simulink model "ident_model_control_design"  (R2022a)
settings: Solver=VariableStepAuto  StartTime=0.0  StopTime=tfin  RelTol=1e-3
undefined symbols (not defined in the file or in its folder): magnitude
libraries: cstblocks x5, mpclib x2, slpidlib x1, ctrlSharedLib x1

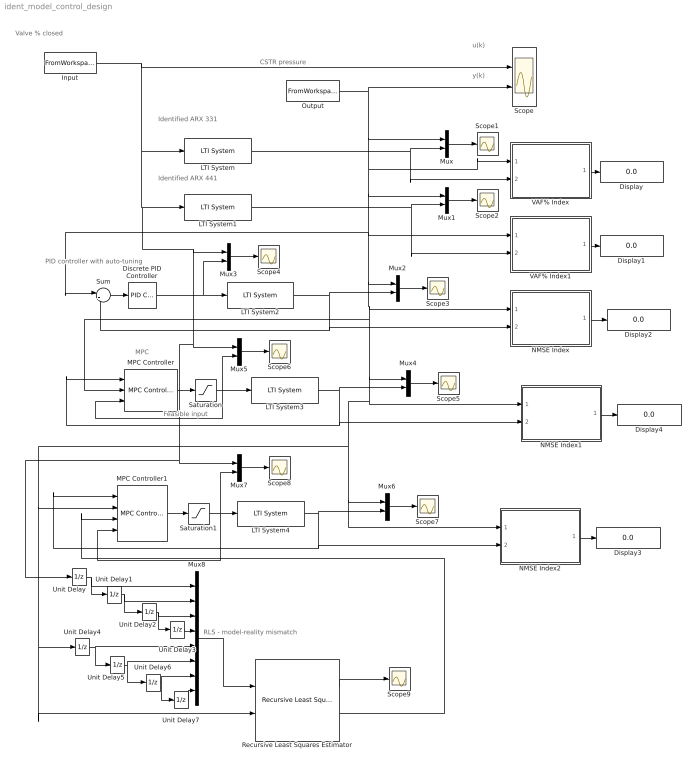
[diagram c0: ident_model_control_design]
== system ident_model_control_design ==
  note: RLS - model-reality mismatch
  note: Feasible input
  note: PID controller with auto-tuning
  note: Identified ARX 441
  note: Identified ARX 331
  note: y(k)
  note: u(k)
  note: CSTR pressure
  note: Valve % closed
  note: MPC
  Discrete PID Controller : slpidlib/PID Controller  Controller=PID  Form=Parallel  TimeDomain=Discrete-time  UseExternalTs=off  SampleTime=5  IntegratorMethod=Forward Euler  FilterMethod=Backward Euler  ControllerParametersSource=internal  P=34.9781098991711  I=1.59717324757153  UseKiTs=off  D=0  N=100  UseFilter=on  TunerSelectOption=Transfer Function Based (PID Tuner App)  InitialConditionSource=internal  InitialConditionForIntegrator=0  InitialConditionForFilter=0  DifferentiatorICPrevScaledInput=0  ExternalReset=none  TrackingMode=off  Kt=1  LimitOutput=off  SatLimitsSource=internal  UpperSaturationLimit=inf  LowerSaturationLimit=-inf  LinearizeAsGain=off  AntiWindupMode=none  Kb=1  POutMin=[]  POutMax=[]  IOutMin=[]  IOutMax=[]  DOutMin=[]  DOutMax=[]  NOutMin=[]  NOutMax=[]  SumOutMin=[]  SumOutMax=[]  SaturationOutMin=[]  SaturationOutMax=[]  PParamMin=[]  PParamMax=[]  IParamMin=[]  IParamMax=[]  DParamMin=[]  DParamMax=[]  NParamMin=[]  NParamMax=[]  KbParamMin=[]  KbParamMax=[]  KtParamMin=[]  KtParamMax=[]  KbOutMin=[]  KbOutMax=[]  KtOutMin=[]  KtOutMax=[]  IntegratorOutMin=[]  IntegratorOutMax=[]  FilterOutMin=[]  FilterOutMax=[]  SumI1OutMin=[]  SumI1OutMax=[]  SumI2OutMin=[]  SumI2OutMax=[]  SumI3OutMin=[]  SumI3OutMax=[]  SumI4OutMin=[]  SumI4OutMax=[]  SumDOutMin=[]  SumDOutMax=[]  DifferentiatorOutMin=[]  DifferentiatorOutMax=[]  FilterDiffOutCoefMin=[]  FilterDiffOutCoefMax=[]  ReciprocalOutMin=[]  ReciprocalOutMax=[]  SumDenOutMin=[]  SumDenOutMax=[]  SumNumOutMin=[]  SumNumOutMax=[]  DivideOutMin=[]  DivideOutMax=[]  UdiffTsProdOutMin=[]  UdiffTsProdOutMax=[]  NTsProdOutMin=[]  NTsProdOutMax=[]  UintegralTsProdOutMin=[]  UintegralTsProdOutMax=[]  UngainTsProdOutMin=[]  UngainTsProdOutMax=[]  ClampingZeroOutDataTypeStr=Inherit: Inherit via back propagation  ClampingZeroOutMin=[]  ClampingZeroOutMax=[]  FilterDenConstantOutDataTypeStr=Inherit: Inherit via back propagation  FilterDenConstantOutMin=[]  FilterDenConstantOutMax=[]  PCopyOutDataTypeStr=Inherit: Inherit via back propagation  PCopyOutMin=[]  PCopyOutMax=[]  NCopyOutDataTypeStr=Inherit: Inherit via back propagation  NCopyOutMin=[]  NCopyOutMax=[]  IntegratorContinuousStateAttributes=''  IntegratorStateMustResolveToSignalObject=off  IntegratorRTWStateStorageClass=Auto  FilterContinuousStateAttributes=''  FilterStateMustResolveToSignalObject=off  FilterRTWStateStorageClass=Auto  ParallelPVariant=InternalParameters  IdealPVariant=Disabled  IVariant=InternalParameters  DVariant=InternalParameters  IntegratorVariant=Discrete  SatVariant=Disabled  AWVariant=Passthrough  PCopyVariant=Disabled  TRVariant=Disabled  FdbkBlocksVariant=Forward  IdealPFdbkVariant=Disabled  SatFdbkVariant=Disabled  DerivativeFilterVariant=BackwardEulerFilter  NVariant=InternalParameters  NCopyVariant=InternalParameters  FilterICVariant=InternalICsFilter  IntegratorICVariant=InternalICs  ExternalResetVariant=Disabled  TRSumVariant=Passthrough  SumFdbkVariant=Disabled  SumVariant=Sum_PID  TsampFilterVariant=InternalTs  TsampNgainVariant=Passthrough  TsampIntegralVariant=Passthrough  ExternalSaturationOutDataTypeStr=Inherit: Same as second input  aMode=0
  Display{,1..4} (5 alike) : Display
  Input : FromWorkspace  VariableName=[tsim U]  SampleTime=5
  LTI System : cstblocks/LTI System  sys=arx331  IC=[]
  LTI System{1..4} (4 alike) : cstblocks/LTI System  sys=arx441  IC=[]
  MPC Controller : mpclib/MPC Controller  SCDEnableBlockLinearizationSpecification=on  mpcobj=mpc1  is_multiple=0  enable_value=0  return_u0=off  updateMPCinCallerWorkspace=on  md_inport=off  mv_inport=on  uref_inport=off  return_cost=off  return_mvseq=off  return_qpstatus=off  return_xseq=off  return_state=off  return_ovseq=off  state_inport=off  umin_inport=off  umax_inport=off  ymin_inport=off  ymax_inport=off  cc_inport=off  ywt_inport=off  uwt_inport=off  duwt_inport=off  rhoeps_inport=off  pm_inport=off  MaximumP=10  HorizonChoice=FixedHorizon  n_ts=5  n_p=25  n_mv=1  n_md=1  n_ud=0  n_mo=1  n_uo=0  BlockDataType=double  SampleTimeInherited=off  switch_inport=off
  MPC Controller1 : mpclib/MPC Controller  SCDEnableBlockLinearizationSpecification=on  mpcobj=mpc1  is_multiple=0  enable_value=0  return_u0=off  updateMPCinCallerWorkspace=on  md_inport=on  mv_inport=on  uref_inport=off  return_cost=off  return_mvseq=off  return_qpstatus=off  return_xseq=off  return_state=off  return_ovseq=off  state_inport=off  umin_inport=off  umax_inport=off  ymin_inport=off  ymax_inport=off  cc_inport=off  ywt_inport=off  uwt_inport=off  duwt_inport=off  rhoeps_inport=off  pm_inport=off  MaximumP=10  HorizonChoice=FixedHorizon  n_ts=5  n_p=25  n_mv=1  n_md=1  n_ud=0  n_mo=1  n_uo=0  BlockDataType=double  SampleTimeInherited=off  switch_inport=off
  Mux{,1..7} (8 alike) : Mux  Inputs=2
  Mux8 : Mux  Inputs=8
  NMSE Index : Subsystem
  NMSE Index1 : Subsystem
  NMSE Index2 : Subsystem
  Output : FromWorkspace  VariableName=[tsim Y]  SampleTime=5
  Recursive Least Squares Estimator : ctrlSharedLib/Recursive Least Squares Estimator  InitialEstimateSource=None  InitialParameterData=8  P0=1e4  InitialRegressors=0  InitialOutputs=0  History=Infinite  WindowLength=200  EstimationMethod=Forgetting Factor  AdaptationParameter=0.97  HasTimeVaryingAdaptationParameter=off  NormalizationBias=eps  OutputError=on  OutputP=off  AddEnablePort=off  InputProcessing=Sample-based  Ts=5
  Saturation : Saturate  UpperLimit=100  LowerLimit=0
  Saturation1 : Saturate  UpperLimit=100  LowerLimit=0
  Scope : Scope  NumInputPorts=2
  Scope{1..9} (9 alike) : Scope
  Sum : Sum  Inputs=|+-
  Unit Delay{,1..7} (8 alike) : UnitDelay  SampleTime=-1  HasFrameUpgradeWarning=on
  VAF% Index : Subsystem
  VAF% Index1 : Subsystem
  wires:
  LTI System/1 -> VAF% Index/2(y_prev), Mux/2
  Mux/1 -> Scope1/1
  LTI System1/1 -> VAF% Index1/2(y_prev), Mux1/2
  Mux1/1 -> Scope2/1
  VAF% Index/1(VAF%) -> Display/1
  VAF% Index1/1(VAF%) -> Display1/1
  Discrete PID Controller/1 -> Mux3/2, LTI System2/1
  Sum/1 -> Discrete PID Controller/1
  LTI System2/1 -> Mux2/2, NMSE Index/2(y_prev), Sum/2
  Mux2/1 -> Scope3/1
  Mux3/1 -> Scope4/1
  NMSE Index/1(NMSE) -> Display2/1
  NMSE Index1/1(NMSE) -> Display4/1
  Mux4/1 -> Scope5/1
  LTI System3/1 -> Mux4/2, MPC Controller/1, NMSE Index1/2(y_prev)
  Mux5/1 -> Scope6/1
  MPC Controller/1 -> Saturation/1
  Saturation/1 -> LTI System3/1, MPC Controller/3, Mux5/2
  Saturation1/1 -> MPC Controller1/4, Mux7/2, LTI System4/1
  LTI System4/1 -> Mux6/2, NMSE Index2/2(y_prev), MPC Controller1/1
  NMSE Index2/1(NMSE) -> Display3/1
  Mux6/1 -> Scope7/1
  Mux7/1 -> Scope8/1
  MPC Controller1/1 -> Saturation1/1
  Unit Delay/1 -> Mux8/1, Unit Delay1/1
  Unit Delay1/1 -> Mux8/2, Unit Delay2/1
  Unit Delay2/1 -> Mux8/3, Unit Delay3/1
  Unit Delay3/1 -> Mux8/4
  Input/1 -> Mux5/1, Unit Delay/1, Mux7/1, Mux3/1, LTI System1/1, LTI System/1, Scope/1
  Unit Delay5/1 -> Mux8/6, Unit Delay6/1
  Output/1 -> VAF% Index/1(y_mis), MPC Controller/2, Mux4/1, Unit Delay4/1, Recursive Least Squares Estimator/2, MPC Controller1/2, Mux6/1, NMSE Index2/1(y_mis), NMSE Index1/1(y_mis), NMSE Index/1(y_mis), Mux2/1, Sum/1, VAF% Index1/1(y_mis), Mux1/1, Mux/1, Scope/2
  Unit Delay4/1 -> Mux8/5, Unit Delay5/1
  Unit Delay6/1 -> Mux8/7, Unit Delay7/1
  Unit Delay7/1 -> Mux8/8
  Mux8/1 -> Recursive Least Squares Estimator/1
  Recursive Least Squares Estimator/1 -> Scope9/1
  Recursive Least Squares Estimator/2 -> MPC Controller1/3

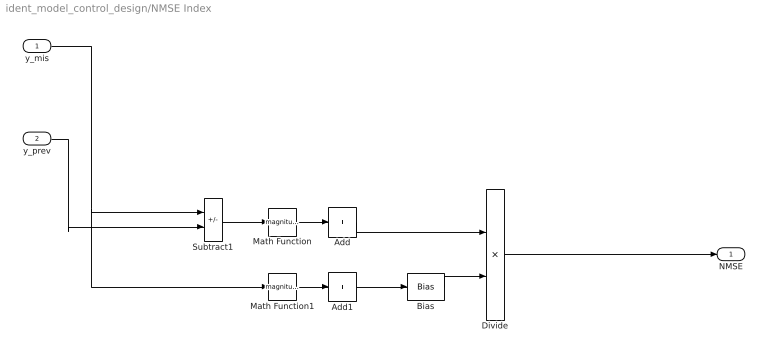
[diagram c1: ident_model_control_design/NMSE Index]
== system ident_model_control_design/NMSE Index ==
  y_mis : Inport
  y_prev : Inport  Port=2
  Add : Sum  Inputs=+
  Add1 : Sum  Inputs=+
  Bias : Bias  Bias=1e-7
  Divide : Product  Inputs=*/
  Math Function : Math  Operator=magnitude^2
  Math Function1 : Math  Operator=magnitude^2
  Subtract1 : Sum  Inputs=+-
  NMSE : Outport
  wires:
  Math Function/1 -> Add/1
  Bias/1 -> Divide/2
  y_mis/1 -> Math Function1/1, Subtract1/1
  Add1/1 -> Bias/1
  Math Function1/1 -> Add1/1
  Subtract1/1 -> Math Function/1
  Add/1 -> Divide/1
  y_prev/1 -> Subtract1/2
  Divide/1 -> NMSE/1

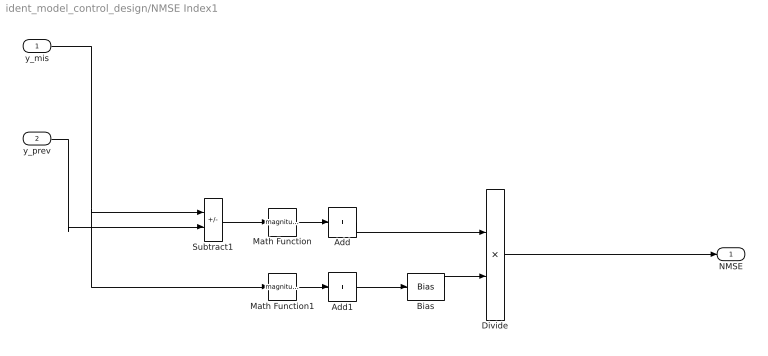
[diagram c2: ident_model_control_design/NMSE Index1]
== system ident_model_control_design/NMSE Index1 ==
  y_mis : Inport
  y_prev : Inport  Port=2
  Add : Sum  Inputs=+
  Add1 : Sum  Inputs=+
  Bias : Bias  Bias=1e-7
  Divide : Product  Inputs=*/
  Math Function : Math  Operator=magnitude^2
  Math Function1 : Math  Operator=magnitude^2
  Subtract1 : Sum  Inputs=+-
  NMSE : Outport
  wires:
  Math Function/1 -> Add/1
  Bias/1 -> Divide/2
  y_mis/1 -> Math Function1/1, Subtract1/1
  Add1/1 -> Bias/1
  Math Function1/1 -> Add1/1
  Subtract1/1 -> Math Function/1
  Add/1 -> Divide/1
  y_prev/1 -> Subtract1/2
  Divide/1 -> NMSE/1

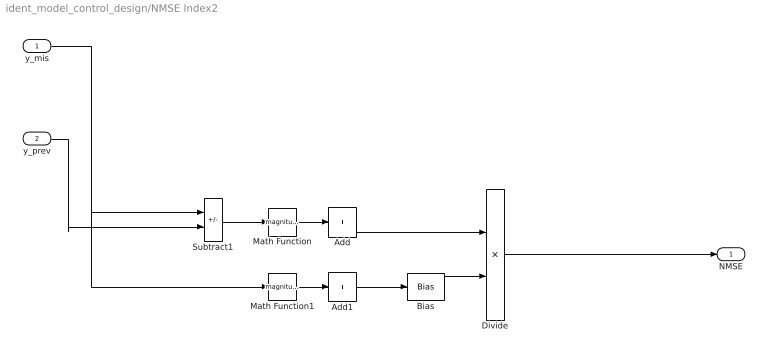
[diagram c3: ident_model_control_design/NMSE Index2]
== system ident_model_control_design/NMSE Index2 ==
  y_mis : Inport
  y_prev : Inport  Port=2
  Add : Sum  Inputs=+
  Add1 : Sum  Inputs=+
  Bias : Bias  Bias=1e-7
  Divide : Product  Inputs=*/
  Math Function : Math  Operator=magnitude^2
  Math Function1 : Math  Operator=magnitude^2
  Subtract1 : Sum  Inputs=+-
  NMSE : Outport
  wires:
  Math Function/1 -> Add/1
  Bias/1 -> Divide/2
  y_mis/1 -> Math Function1/1, Subtract1/1
  Add1/1 -> Bias/1
  Math Function1/1 -> Add1/1
  Subtract1/1 -> Math Function/1
  Add/1 -> Divide/1
  y_prev/1 -> Subtract1/2
  Divide/1 -> NMSE/1

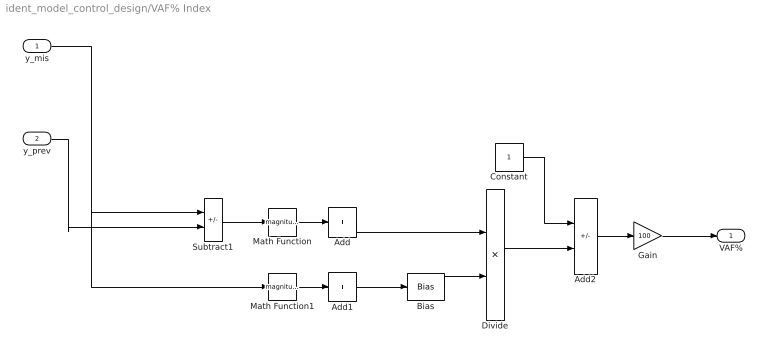
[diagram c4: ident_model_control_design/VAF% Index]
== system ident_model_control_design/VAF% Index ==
  y_mis : Inport
  y_prev : Inport  Port=2
  Add : Sum  Inputs=+
  Add1 : Sum  Inputs=+
  Add2 : Sum  Inputs=+-
  Bias : Bias  Bias=1e-7
  Constant : Constant
  Divide : Product  Inputs=*/
  Gain : Gain  Gain=100
  Math Function : Math  Operator=magnitude^2
  Math Function1 : Math  Operator=magnitude^2
  Subtract1 : Sum  Inputs=+-
  VAF% : Outport
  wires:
  Add2/1 -> Gain/1
  Math Function/1 -> Add/1
  Bias/1 -> Divide/2
  y_mis/1 -> Math Function1/1, Subtract1/1
  Add1/1 -> Bias/1
  Math Function1/1 -> Add1/1
  Subtract1/1 -> Math Function/1
  Constant/1 -> Add2/1
  Divide/1 -> Add2/2
  Add/1 -> Divide/1
  y_prev/1 -> Subtract1/2
  Gain/1 -> VAF%/1

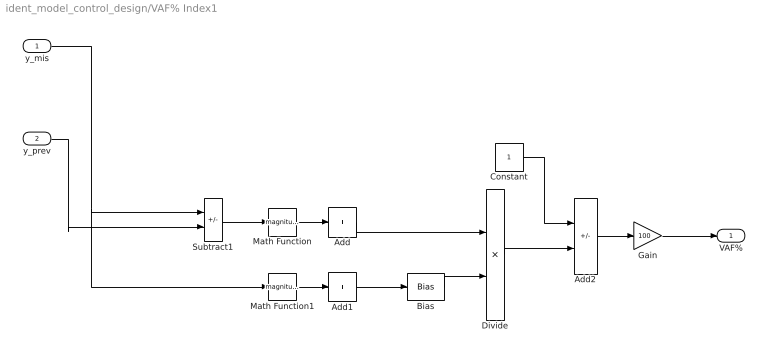
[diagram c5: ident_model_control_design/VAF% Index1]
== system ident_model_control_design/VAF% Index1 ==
  y_mis : Inport
  y_prev : Inport  Port=2
  Add : Sum  Inputs=+
  Add1 : Sum  Inputs=+
  Add2 : Sum  Inputs=+-
  Bias : Bias  Bias=1e-7
  Constant : Constant
  Divide : Product  Inputs=*/
  Gain : Gain  Gain=100
  Math Function : Math  Operator=magnitude^2
  Math Function1 : Math  Operator=magnitude^2
  Subtract1 : Sum  Inputs=+-
  VAF% : Outport
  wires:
  Add2/1 -> Gain/1
  Math Function/1 -> Add/1
  Bias/1 -> Divide/2
  y_mis/1 -> Math Function1/1, Subtract1/1
  Add1/1 -> Bias/1
  Math Function1/1 -> Add1/1
  Subtract1/1 -> Math Function/1
  Constant/1 -> Add2/1
  Divide/1 -> Add2/2
  Add/1 -> Divide/1
  y_prev/1 -> Subtract1/2
  Gain/1 -> VAF%/1
